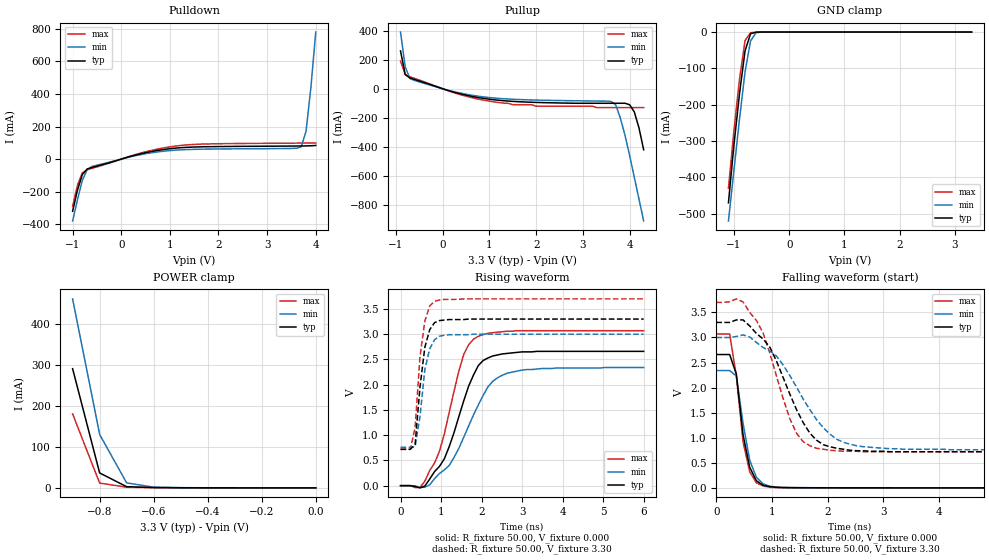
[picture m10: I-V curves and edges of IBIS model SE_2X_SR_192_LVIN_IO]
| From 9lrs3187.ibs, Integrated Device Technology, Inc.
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|   Model SE_2X_SR_192_LVIN_IO
[Model]   SE_2X_SR_192_LVIN_IO
Model_type   I/O
Polarity   Inverting
Enable   Active-High
Vinl =   0.35V
Vinh =   0.7V
Vmeas =   1.50V
Cref =   5.00pF
Rref =  50.000
Vref =   1.50V
C_comp   3.40pF   2.85pF   3.95pF
[Temperature Range]   27.00   70.00   0.000
[Voltage Range]   3.30V   3.00V   3.70V
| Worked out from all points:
|   slope of the pulldown table from 0 to 0.495 V, typ, clamps not added: 12.7 ohm
|   slope of the pullup table from 0 to 0.495 V, typ, clamps not added: 11.3 ohm
|   GND clamp passes 1 mA (typ) near -0.61 V on its own axis
|   POWER clamp passes 1 mA (typ) near -0.61 V on its own axis
|   rising waveform, R_fixture 50.00, V_fixture 0.000: 20-80 % time 685ps typ, 847ps min, 582ps max; typ from 0 V to 2.66 V
|   rising waveform, R_fixture 50.00, V_fixture 3.30: 20-80 % time 211ps typ, 226ps min, 199ps max; typ from 0.72 V to 3.3 V
|   falling waveform, R_fixture 50.00, V_fixture 0.000: 20-80 % time 203ps typ, 223ps min, 213ps max; typ from 2.66 V to 0 V
|   falling waveform, R_fixture 50.00, V_fixture 3.30: 20-80 % time 625ps typ, 782ps min, 513ps max; typ from 3.3 V to 0.72 V
[Pulldown]
| voltage   I(typ)   I(min)   I(max)
|  -3.30   -4.15A   -4.00A   -4.25A
|  -3.10   -3.81A   -3.68A   -3.90A
|  -2.90   -3.47A   -3.36A   -3.55A
|  -2.70   -3.13A   -3.04A   -3.19A
|  -2.50   -2.79A   -2.72A   -2.84A
|  -2.30   -2.46A   -2.40A   -2.49A
|  -2.10   -2.12A   -2.08A   -2.14A
|  -1.90   -1.78A   -1.77A   -1.79A
|  -1.70   -1.45A   -1.45A   -1.45A
|  -1.50   -1.12A   -1.14A   -1.10A
-1V       -320mA     -380mA     -290mA
-900mV    -190mA     -250mA     -160mA
-800mV    -94.69mA   -130mA     -84.74mA
-700mV    -60.71mA   -64.73mA   -65.52mA
-600mV    -51.06mA   -45.2mA    -56.5mA
400mV     32.6mA     27.52mA    37.03mA
1.2V      69.5mA     56.57mA    82.87mA
3.5V      80.08mA    65.45mA    97.87mA
3.7V      80.56mA    75.12mA    98.32mA
3.8V      80.96mA    170mA      98.58mA
3.9V      81.72mA    440mA      98.88mA
4V        83.73mA    780mA      99.22mA
|   4.10   0.11A   1.16A   99.62mA
|   4.20   0.31A   1.55A   0.10A
|   4.30   0.66A   1.95A   0.10A
|   4.50   1.46A   2.77A   0.11A
|   4.70   2.32A   3.59A   0.58A
|   4.90   3.19A   4.43A   1.41A
|   5.10   4.07A   5.27A   2.30A
|   5.30   4.96A   6.11A   3.20A
|   5.50   5.85A   6.96A   4.12A
|   5.70   6.75A   7.81A   5.04A
|   5.90   7.64A   8.66A   5.97A
|   6.10   8.54A   9.51A   6.89A
|   6.60   10.80A   11.65A   9.23A
[Pullup]
| voltage   I(typ)   I(min)   I(max)
|  -3.30   10.68A   10.27A   10.94A
|  -3.10   9.78A   9.42A   10.01A
|  -2.90   8.88A   8.57A   9.08A
|  -2.70   7.99A   7.73A   8.16A
|  -2.50   7.09A   6.88A   7.23A
|  -2.30   6.20A   6.04A   6.30A
|  -2.10   5.31A   5.20A   5.38A
|  -1.90   4.42A   4.36A   4.46A
|  -1.70   3.54A   3.53A   3.55A
|  -1.50   2.67A   2.70A   2.64A
|  -1.00   0.59A   0.73A   0.50A
-900mV    260mA      390mA      190mA
-800mV    98.09mA    150mA      96.73mA
-700mV    74.34mA    69.92mA    82.79mA
-600mV    63.81mA    56.49mA    71.52mA
500mV     -44.25mA   -37.82mA   -51.47mA
1.5V      -86.95mA   -72.42mA   -110mA
3.5V      -100mA     -85.41mA   -130mA
3.7V      -100mA     -110mA     -130mA
3.9V      -100mA     -320mA     -130mA
4.1V      -160mA     -610mA     -130mA
4.2V      -270mA     -760mA     -130mA
4.3V      -420mA     -910mA     -130mA
|   4.50   -0.73A   -1.22A   -0.15A
|   4.70   -1.06A   -1.54A   -0.40A
|   4.90   -1.39A   -1.85A   -0.72A
|   5.10   -1.72A   -2.17A   -1.06A
|   5.30   -2.06A   -2.49A   -1.40A
|   5.50   -2.39A   -2.81A   -1.75A
|   5.70   -2.73A   -3.13A   -2.10A
|   5.90   -3.07A   -3.45A   -2.45A
|   6.10   -3.41A   -3.77A   -2.80A
|   6.60   -4.26A   -4.58A   -3.68A
[GND_clamp]
| voltage   I(typ)   I(min)   I(max)
|  -3.30   -4.15A   -4.00A   -4.25A
|  -3.20   -3.98A   -3.84A   -4.07A
|  -3.10   -3.81A   -3.68A   -3.90A
|  -3.00   -3.64A   -3.52A   -3.72A
|  -2.90   -3.47A   -3.36A   -3.55A
|  -2.80   -3.30A   -3.20A   -3.37A
|  -2.70   -3.13A   -3.04A   -3.19A
|  -2.60   -2.96A   -2.88A   -3.02A
|  -2.50   -2.79A   -2.72A   -2.84A
|  -2.40   -2.62A   -2.56A   -2.67A
|  -2.30   -2.45A   -2.40A   -2.49A
|  -2.20   -2.29A   -2.24A   -2.32A
|  -2.10   -2.12A   -2.08A   -2.14A
|  -2.00   -1.95A   -1.92A   -1.97A
|  -1.90   -1.78A   -1.76A   -1.79A
|  -1.80   -1.61A   -1.61A   -1.62A
|  -1.70   -1.45A   -1.45A   -1.45A
|  -1.60   -1.28A   -1.29A   -1.27A
|  -1.50   -1.12A   -1.14A   -1.10A
|  -1.40   -0.95A   -0.98A   -0.93A
|  -1.30   -0.79A   -0.83A   -0.76A
|  -1.20   -0.63A   -0.67A   -0.59A
-1.1V     -470mA     -520mA     -430mA
-1V       -310mA     -380mA     -270mA
-900mV    -170mA     -240mA     -130mA
-800mV    -52.1mA    -110mA     -23.59mA
-700mV    -4.69mA    -24.29mA   -1.84mA
-600mV    -430uA     -1.9mA     -210uA
-400mV    -1.76uA    -10.19uA   -470nA
3.3V      150pA      24.14uA    -330pA
[POWER_clamp]
| voltage   I(typ)   I(min)   I(max)
|  -3.30   13.34A   12.83A   13.67A
|  -3.20   12.78A   12.30A   13.09A
|  -3.10   12.22A   11.77A   12.51A
|  -3.00   11.66A   11.24A   11.93A
|  -2.90   11.10A   10.71A   11.35A
|  -2.80   10.54A   10.18A   10.77A
|  -2.70   9.98A   9.66A   10.19A
|  -2.60   9.42A   9.13A   9.61A
|  -2.50   8.86A   8.60A   9.03A
|  -2.40   8.31A   8.07A   8.46A
|  -2.30   7.75A   7.54A   7.88A
|  -2.20   7.19A   7.02A   7.30A
|  -2.10   6.64A   6.49A   6.73A
|  -2.00   6.08A   5.97A   6.15A
|  -1.90   5.53A   5.45A   5.58A
|  -1.80   4.97A   4.92A   5.00A
|  -1.70   4.42A   4.40A   4.43A
|  -1.60   3.88A   3.89A   3.86A
|  -1.50   3.33A   3.37A   3.30A
|  -1.40   2.79A   2.86A   2.74A
|  -1.30   2.25A   2.35A   2.18A
|  -1.20   1.72A   1.85A   1.63A
|  -1.10   1.21A   1.37A   1.10A
|  -1.00   0.72A   0.90A   0.60A
-900mV    290mA      460mA      180mA
-800mV    36.29mA    130mA      11.65mA
-700mV    2.83mA     12.05mA    1.52mA
-600mV    760uA      1.75mA     430uA
-500mV    190uA      510uA      90.12uA
-400mV    36.78uA    130uA      14.36uA
-300mV    5.51uA     24.14uA    1.75uA
-200mV    600nA      3.69uA     140nA
-100mV    40.72nA    380nA      6.97nA
0V        150pA      200pA      160pA
[Ramp]
| variable   typ   min   max
dV/dt_r   1.60/0.68n   1.40/0.84n   1.84/0.57n
dV/dt_f   1.55/0.62n   1.34/0.77n   1.79/0.50n
R_load = 50.00
[Rising Waveform]
R_fixture = 50.00
V_fixture = 0.000
V_fixture_min = 0.000
V_fixture_max = 0.000
| time   V(typ)   V(min)   V(max)
0s        0V         1.34uV     0V
480ps     -43.38mV   -36.81mV   -36.84mV
840ps     280mV      140mV      450mV
1.08ns    530mV      310mV      1.02V
1.56ns    1.68V      960mV      2.6V
1.8ns     2.19V      1.4V       2.9V
1.92ns    2.38V      1.6V       2.96V
2.16ns    2.53V      1.96V      3.02V
2.64ns    2.62V      2.23V      3.06V
6ns       2.66V      2.34V      3.07V
[Rising Waveform]
R_fixture = 50.00
V_fixture = 3.30
V_fixture_min = 3.00
V_fixture_max = 3.70
| time   V(typ)   V(min)   V(max)
0s        720mV      760mV      720mV
240ps     720mV      760mV      720mV
360ps     820mV      770mV      1.15V
480ps     1.95V      1.37V      2.55V
600ps     2.74V      2.3V       3.26V
720ps     3.09V      2.71V      3.56V
840ps     3.23V      2.89V      3.65V
960ps     3.27V      2.96V      3.68V
1.2ns     3.29V      2.99V      3.69V
6ns       3.3V       3V         3.7V
[Falling Waveform]
R_fixture = 50.00
V_fixture = 0.000
V_fixture_min = 0.000
V_fixture_max = 0.000
| time   V(typ)   V(min)   V(max)
0s        2.66V      2.34V      3.07V
240ps     2.66V      2.34V      3.07V
360ps     2.27V      2.23V      2.23V
480ps     1.06V      1.29V      920mV
600ps     410mV      550mV      320mV
720ps     140mV      210mV      100mV
840ps     52.27mV    79mV       37.5mV
960ps     23.77mV    32.48mV    11.83mV
1.32ns    3.61mV     5.56mV     2.9mV
6ns       0V         1.85uV     0V
[Falling Waveform]
R_fixture = 50.00
V_fixture = 3.30
V_fixture_min = 3.00
V_fixture_max = 3.70
| time   V(typ)   V(min)   V(max)
0s        3.3V       3V         3.7V
360ps     3.35V      3.02V      3.77V
720ps     3.08V      2.9V       3.34V
960ps     2.81V      2.73V      2.69V
1.32ns    1.87V      2.24V      1.38V
1.44ns    1.56V      2.01V      1.09V
1.68ns    1.09V      1.56V      840mV
2.04ns    820mV      1.07V      750mV
2.52ns    740mV      840mV      730mV
6ns       720mV      760mV      720mV
